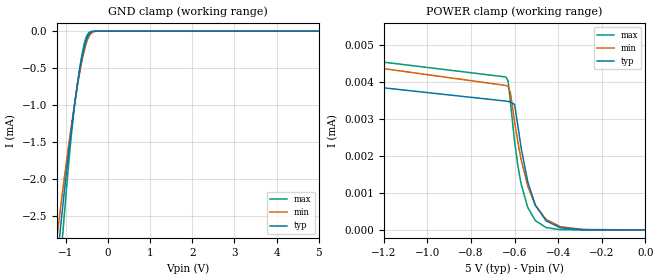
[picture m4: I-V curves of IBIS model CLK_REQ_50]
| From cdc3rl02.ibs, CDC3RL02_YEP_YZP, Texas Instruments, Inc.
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[Model]   CLK_REQ_50
Model_type  Input
Vinl=0.5
Vinh=1.3
| variable   typ   min   max
C_comp   1.90pF   1.34pF   2.13pF
[Temperature Range]   40   100   -40
| Ambient temperature   25   85   -40
[Voltage range]   5   4.5   5.5
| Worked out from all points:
|   GND clamp passes 1 mA (typ) near -0.79 V on its own axis
[GND Clamp]
| CLK_REQ_50
|   Voltage   I(typ)   I(min)   I(max)
-5V       -31.28mA   -27.04mA   -38.32mA
-1.2V     -3.098mA   -2.763mA   -3.7mA
-1.16V    -2.871mA   -2.572mA   -3.403mA
-1.12V    -2.648mA   -2.385mA   -3.11mA
-1.06V    -2.322mA   -2.111mA   -2.682mA
-865mV    -1.34mA    -1.281mA   -1.409mA
-725mV    -735.5uA   -756.9uA   -731uA
-565mV    -235.3uA   -278.7uA   -185.2uA
-495mV    -98.22uA   -138.3uA   -59.08uA
-420mV    -23.68uA   -47.86uA   -9.357uA
-240mV    -169nA     -976.9nA   -10.01nA
5V        180.8pA    611.1nA    113.1pA
[POWER Clamp]
| CLK_REQ_50
|   Voltage   I(typ)   I(min)   I(max)
-5V       1.186mA    1.105mA    1.634mA
-2.18V    54.15uA    5.416uA    168.3uA
-1.96V    5.427uA    4.954uA    63.04uA
-1.9V     4.407uA    4.908uA    37.49uA
-1.76V    4.189uA    4.8uA      5.534uA
-1.66V    4.126uA    4.723uA    4.853uA
-640mV    3.476uA    3.898uA    4.127uA
-600mV    3.383uA    2.916uA    2.374uA
-570mV    2.211uA    1.893uA    1.235uA
-505mV    669.7nA    664.8nA    251.5nA
-390mV    59.4nA     87.78nA    8.687nA
0V        0A         0A         0A
